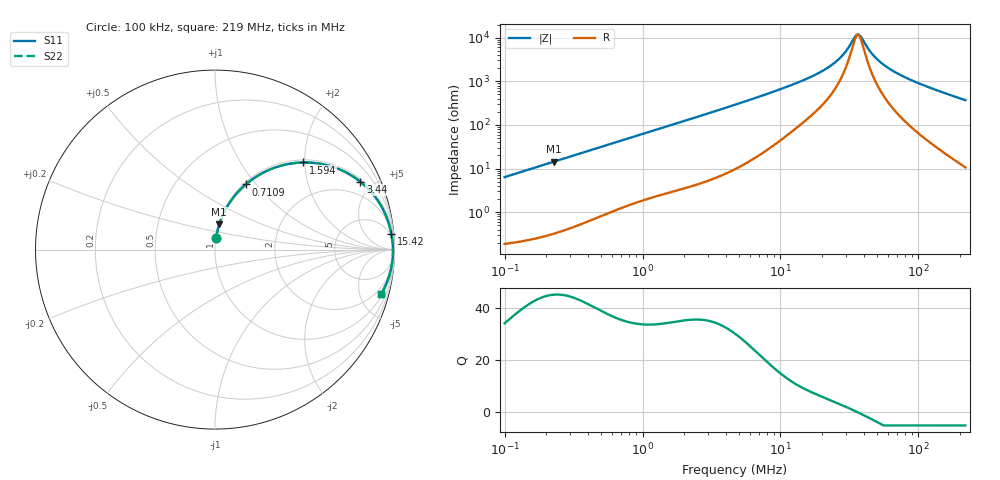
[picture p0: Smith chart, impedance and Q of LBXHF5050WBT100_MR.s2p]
! LBXHF5050WBT100_MR  S-PARAMETER MODEL  ( General Type )
! Model Generated by TAIYO YUDEN Corporation (http://www.ty-top.com)
! Version 1.0
! TAIYO YUDEN Control No. 210719NI43SB-FBB
! Copyright(c) 2021 TAIYO YUDEN CO.,LTD. All Rights Reserved.
! Product Description (link to TY-COMPAS)
! https://ds.yuden.co.jp/TYCOMPAS/or/detail?pn=LBXHF5050WBT100MMR&u=M
! Products Name : Inductors
! Characteristics :
!  Inductance : 10 uH , SRF(min) : 25 MHz , DC Resistance(max) : 0.1272 Ohm
!  Rated Current : Saturation :1500 mA , Temp Rise : 1100 mA
!  Case Size : 5.0 x 5.0 / 0.197 x 0.197 [mm/inch] , Thickness : 2.2 / 0.087 [mm/inch]
!  (Conditions: Temperature = 25 degC , DC Bias Current/Voltage = 0A / 0V)
! External Node Assignments :
!  1  o---GGG---o  2
! GND o---------o GND
! Frequency Range : 0.1MHz  -  218.972167MHz  [ 402 STEP ]
# MHz S RI R 50
! Freq[MHz].  S11 Real  S11 Imag  S21 Real  S21 Imag  S12 Real  S12 Imag  S22 Real  S22 Imag
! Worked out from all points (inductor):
!   401 points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, 100 kHz to 219 MHz, reference 50 ohm
!   read as one part in series: L = 10.1 uH near 103.9 kHz
!   highest Q = 44.9 at 228.6 kHz (marker M1), where L = 10.1 uH
!   self-resonance near 35.93 MHz
!   S11 on the Smith chart (normalised r, x): 100 kHz: 1.00, +0.13; 710.9 kHz: 1.03, +0.89; 1.594 MHz: 1.06, +1.96; 3.44 MHz: 1.12, +4.23; 15.42 MHz: 4, +23; 219 MHz: 1.21, -7.38
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0.1  0.00588 0.0631  0.9941 -0.0631  0.9941 -0.0631  0.00588 0.0631
0.228608  0.0236 0.1409  0.9764 -0.1409  0.9764 -0.1409  0.0236 0.1409
0.362673  0.0544 0.2153  0.9456 -0.2153  0.9456 -0.2153  0.0544 0.2153
0.710885  0.1718 0.3633  0.8282 -0.3633  0.8282 -0.3633  0.1718 0.3633
1.315317  0.4002 0.4753  0.5998 -0.4753  0.5998 -0.4753  0.4002 0.4753
1.59419  0.4908 0.4855  0.5092 -0.4855  0.5092 -0.4855  0.4908 0.4855
2.2535  0.6526 0.4622  0.3474 -0.4622  0.3474 -0.4622  0.6526 0.4622
3.440162  0.8104 0.3776  0.1896 -0.3776  0.1896 -0.3776  0.8104 0.3776
4.770297  0.8895 0.2971  0.1105 -0.2971  0.1105 -0.2971  0.8895 0.2971
9.172305  0.9637 0.1592  0.0363 -0.1592  0.0363 -0.1592  0.9637 0.1592
15.4154  0.9825 0.0851  0.0175 -0.0851  0.0175 -0.0851  0.9825 0.0851
16.97108  0.9845 0.0741  0.0155 -0.0741  0.0155 -0.0741  0.9845 0.0741
21.37574  0.9881 0.0498  0.0119 -0.0498  0.0119 -0.0498  0.9881 0.0498
25.90783  0.99 0.0311  0.00995 -0.0311  0.00995 -0.0311  0.99 0.0311
29.64065  0.9909 0.0187  0.00905 -0.0187  0.00905 -0.0187  0.9909 0.0187
34.5697  0.9915 0.00467  0.00846 -0.00467  0.00846 -0.00467  0.9915 0.00467
36.62254  0.9916 -0.000552  0.00836 0.000552  0.00836 0.000552  0.9916 -0.000552
38.79729  0.9917 -0.00578  0.00832 0.00578  0.00832 0.00578  0.9917 -0.00578
47.93603  0.9913 -0.0253  0.00872 0.0253  0.00872 0.0253  0.9913 -0.0253
61.54953  0.9896 -0.0499  0.0104 0.0499  0.0104 0.0499  0.9896 -0.0499
101.4729  0.9801 -0.1093  0.0199 0.1093  0.0199 0.1093  0.9801 -0.1093
218.9722  0.9255 -0.2486  0.0745 0.2486  0.0745 0.2486  0.9255 -0.2486
